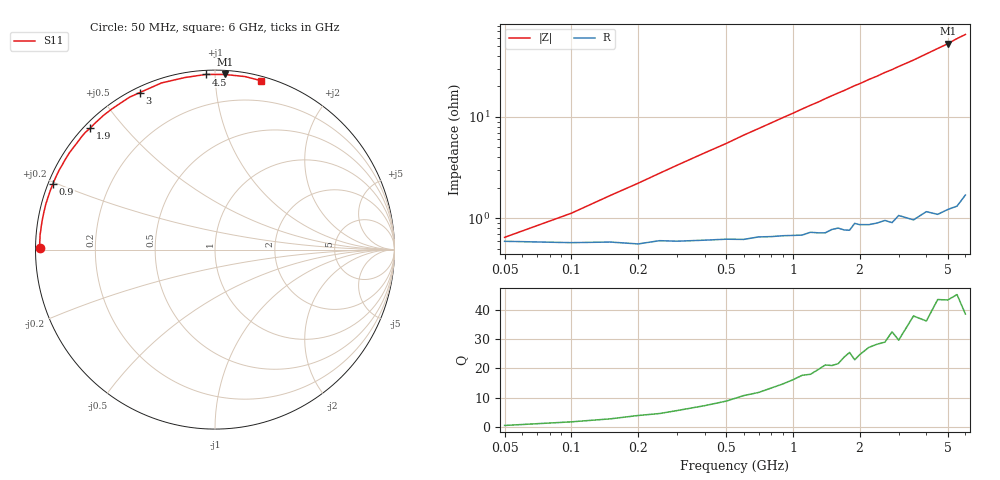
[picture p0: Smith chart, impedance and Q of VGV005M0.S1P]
! Infineon Technologies  Discrete & RF Semiconductors
! BB 831
! Si Tuning Diode in SOD323
! VR =
! S-Parameters:  July  1999
# GHz  S  MA  R  50
!  f  S11
! GHz  MAG  ANG
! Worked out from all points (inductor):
!   34 points, 50 MHz to 6 GHz, reference 50 ohm
!   read as one part to ground: L = 1.72 nH near 200 MHz
!   highest Q = 43.6 at 5 GHz (marker M1), where L = 1.68 nH
!   S11 on the Smith chart (normalised r, x): 50 MHz: 0.01, +0.01; 900 MHz: 0.01, +0.20; 1.9 GHz: 0.02, +0.41; 3 GHz: 0.02, +0.63; 4.5 GHz: 0.02, +0.95; 6 GHz: 0.03, +1.31
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0.05  0.9767 179.4
0.1  0.9774 177.8
0.15  0.9771 176.4
0.2  0.9781 175.1
0.4  0.9763 170.0
0.6  0.9761 165.0
0.8  0.9748 160.2
0.9  0.9745 157.8
1  0.9746 155.5
1.2  0.9732 150.8
1.3  0.9738 148.7
1.4  0.9741 146.3
1.6  0.9719 142.0
1.7  0.9734 140.0
1.8  0.9739 137.8
1.9  0.97 135.7
2  0.9712 133.9
2.2  0.9721 129.8
2.4  0.9719 126.3
2.6  0.9713 122.4
2.8  0.9735 119.2
3  0.9701 115.6
3.5  0.9752 107.8
4  0.9732 100.0
4.5  0.9773 93.0
5  0.9773 86.8
5.5  0.9785 80.1
6  0.9753 74.9
